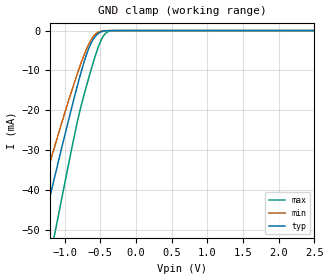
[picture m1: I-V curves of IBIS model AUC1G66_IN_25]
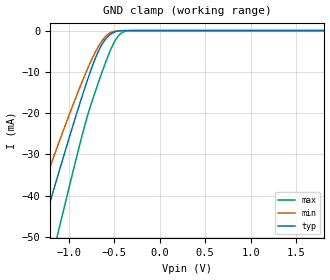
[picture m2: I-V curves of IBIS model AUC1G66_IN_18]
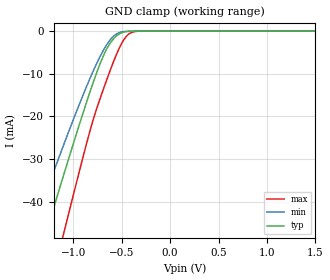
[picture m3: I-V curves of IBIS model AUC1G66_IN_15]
| TEXAS INSTRUMENTS INCORPORATED
| Standard Linear and Logic Group
| IBIS Model of SN74AUC1G66
| SINGLE BILATERAL ANALOG SWITCH
| This file contains package information for the following:
|  SOT 5-pin (DBV) package as [Component] AUC1G66_DBV
|  SOT 5-pin (DCK) package as [Component] AUC1G66_DCK
|  NanoStar WCSP 5-pin (YEA) package as [Component] AUC1G66_YEA
|  NanoFree WCSP 5-pin (YZA) package as [Component] AUC1G66_YZA
| This device can be powered at the following Vccs:
|  2.5 volt Vcc
|  1.8 volt Vcc
|  1.5 volt Vcc
|  1.2 volt Vcc
| This file provides unique models under the [Model Selector] for each Vcc.
| For operation at a specific Vcc, select the appropriate model after each
| [Model Selector] keyword.
[IBIS Ver]   3.2
[Comment char]  |_char
[File Name]   sn74auc1g66.ibs
[File Rev]   1.1 | x_die
[Date]   March 18, 2003
[Source]   Data created from TI-SPICE simulations at TI-SLL.
[Notes]   The following is an IBIS list for the SN74AUC1G66.
   Please contact sllibis@ti.com with questions and
   comments concerning SLL IBIS models.
   - Non-monotonic data due to FET characteristics.
   - C_comp values are taken at a different test condition than
   the Ci/Cio in data sheet.
   - Power-clamp data has been deleted from the input model
   since there is no power-clamp diode.
[Disclaimer] Property of Texas Instruments Incorporated. Unauthorized
   reproduction and/or distribution is strictly prohibited.
   This product is protected under copyright law.
   Created 2003,(C) Copyright 2003, Texas Instruments
   Incorporated, All Rights Reserved
   UNLESS THERE IS A SIGNED, WRITTEN AGREEMENT TO THE
   CONTRARY, TEXAS INSTRUMENTS (TI) IS PROVIDING THE IBIS
   MODELS AND WITHOUT ANY WARRANTY, EXPRESSED OR
   IMPLIED. TI assumes no liability for:
   1) the accuracy of the IBIS models provided to your
   company;
   2) the proper functioning of these IBIS Models in your
   design or for any resulting applications; or
   3) infringement of patents, copyrights or intellectual
   property rights resulting from your use of these IBIS
   models.
   TI provides IBIS Models as a service to our customers.
   You and your company shall not distribute, sell or give
   these models to anyone else without prior written
   permission from TI.
   TI reserves the right to make changes to our products or
   to discontinue any semiconductor product or service
   without notice, and advises our customers to obtain the
   latest version of relevant information to verify, before
   placing orders, that the information being relied on is
   current.
   Please be aware that your receipt and use of the IBIS
   information provided shall serve as acceptance of these
   terms and conditions. If you do not accept these terms,
   you should return or destroy the IBIS models and any
   other accompanying information immediately.
| Component AUC1G66_DBV 5-pin SOT
[Component]   AUC1G66_DBV
[Manufacturer]   Texas Instruments, Inc.
[Package]
|   typ   min   max
R_pkg   2.500e-02   2.100e-02   2.900e-02
L_pkg   1.529e-09   1.312e-09   1.906e-09
C_pkg   1.560e-13   1.100e-13   2.400e-13
[Pin]   signal_name   model_name   R_pin   L_pin   C_pin
1   A   AUC1G66_IO   2.100e-02   1.511e-09   1.440e-13
2   B   AUC1G66_IO   2.300e-02   1.312e-09   1.380e-13
3   GND   GND   2.900e-02   1.906e-09   2.400e-13
4   C   AUC1G66_IN   2.600e-02   1.541e-09   1.500e-13
5   VCC   POWER   2.500e-02   1.374e-09   1.100e-13
| Component AUC1G66_DCK 5-pin SOT
[Component]   AUC1G66_DCK
[Manufacturer]   Texas Instruments, Inc.
[Package]
|   typ   min   max
R_pkg   2.000e-02   1.700e-02   2.500e-02
L_pkg   9.980e-10   8.810e-10   1.069e-09
C_pkg   1.460e-13   1.180e-13   2.050e-13
[Pin]   signal_name   model_name   R_pin   L_pin   C_pin
1   A   AUC1G66_IO   1.900e-02   1.069e-09   1.620e-13
2   B   AUC1G66_IO   1.800e-02   8.810e-10   1.210e-13
3   GND   GND   1.700e-02   1.031e-09   2.050e-13
4   C   AUC1G66_IN   2.000e-02   9.600e-10   1.240e-13
5   VCC   POWER   2.500e-02   1.049e-09   1.180e-13
| Component AUC1G66_YEA 5-pin NanoStar WCSP
[Component]   AUC1G66_YEA
[Manufacturer]   Texas Instruments, Inc.
[Package]
|   typ   min   max
R_pkg   0.001   0.001   0.001
L_pkg   0.021nH   0.021nH   0.021nH
C_pkg   0.046pF   0.045pF   0.047pF
[Pin]   signal_name   model_name   R_pin   L_pin   C_pin
1   A   AUC1G66_IO   0.001   0.021nH   0.046pF
2   B   AUC1G66_IO   0.001   0.021nH   0.047pF
3   GND   GND   0.001   0.021nH   0.046pF
4   C   AUC1G66_IN   0.001   0.021nH   0.045pF
5   VCC   POWER   0.001   0.021nH   0.045pF
| Component AUC1G66_YZA 5-pin NanoFree WCSP
[Component]   AUC1G66_YZA
[Manufacturer]   Texas Instruments, Inc.
[Package]
|   typ   min   max
R_pkg   0.001   0.001   0.001
L_pkg   0.021nH   0.021nH   0.021nH
C_pkg   0.046pF   0.045pF   0.047pF
[Pin]   signal_name   model_name   R_pin   L_pin   C_pin
1   A   AUC1G66_IO   0.001   0.021nH   0.046pF
2   B   AUC1G66_IO   0.001   0.021nH   0.047pF
3   GND   GND   0.001   0.021nH   0.046pF
4   C   AUC1G66_IN   0.001   0.021nH   0.045pF
5   VCC   POWER   0.001   0.021nH   0.045pF
[Series Switch Groups]
| Function Group States
On  1 /   | A<->B(C=HIGH)
Off 1 /   | A<-x->B(C=LOW)
[Series Pin Mapping]   pin_2   model_name   function_table_group
1   2   AUC1G66_IO_25_S   1
| 1   2   AUC1G66_IO_18_S   1
| 1   2   AUC1G66_IO_15_S   1
| 1   2   AUC1G66_IO_12_S   1
| Model AUC1G66_IN
[Model Selector]   AUC1G66_IN
AUC1G66_IN_25   2.5 volt Vcc
AUC1G66_IN_18   1.8 volt Vcc
AUC1G66_IN_15   1.5 volt Vcc
AUC1G66_IN_12   1.2 volt Vcc
| Model AUC1G66_IO
[Model Selector]   AUC1G66_IO
AUC1G66_IO_25   2.5 volt Vcc
AUC1G66_IO_18   1.8 volt Vcc
AUC1G66_IO_15   1.5 volt Vcc
AUC1G66_IO_12   1.2 volt Vcc
| Model AUC1G66_IO_S
[Model Selector]   AUC1G66_IO_S
AUC1G66_IO_25_S   2.5 volt Vcc
AUC1G66_IO_18_S   1.8 volt Vcc
AUC1G66_IO_15_S   1.5 volt Vcc
AUC1G66_IO_12_S   1.2 volt Vcc
[Model]   AUC1G66_IO_25_S
Model_type  Series_switch
| variable   typ   min   max
C_comp   0   0   0
[Temperature Range]   40   100   -40
| Ambient temperature   25   85   -40
[Voltage range]   2.5   2.3   2.7
[On]
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[Off]
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[Model]   AUC1G66_IO_18_S
Model_type  Series_switch
| variable   typ   min   max
C_comp   0   0   0
[Temperature Range]   40   100   -40
| Ambient temperature   25   85   -40
[Voltage range]   1.8   1.65   1.95
[On]
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[Off]
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[Model]   AUC1G66_IO_15_S
Model_type  Series_switch
| variable   typ   min   max
C_comp   0   0   0
[Temperature Range]   40   100   -40
| Ambient temperature   25   85   -40
[Voltage range]   1.5   1.4   1.6
[On]
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[Off]
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[Model]   AUC1G66_IO_12_S
Model_type  Series_switch
| variable   typ   min   max
C_comp   0   0   0
[Temperature Range]   40   100   -40
| Ambient temperature   25   85   -40
[Voltage range]   1.2   1.1   1.3
[On]
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[Off]
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| Models and submodels in the file (12): AUC1G66_IN_25 (Input), AUC1G66_IN_18 (Input), AUC1G66_IN_15 (Input), AUC1G66_IN_12 (Input), AUC1G66_IO_25_S (Series_switch), AUC1G66_IO_25 (Terminator), AUC1G66_IO_18_S (Series_switch), AUC1G66_IO_18 (Terminator), AUC1G66_IO_15_S (Series_switch), AUC1G66_IO_15 (Terminator), AUC1G66_IO_12_S (Series_switch), AUC1G66_IO_12 (Terminator)
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[Model]   AUC1G66_IN_25
Model_type  Input
Vinl=0.7
Vinh=1.7
| variable   typ   min   max
C_comp   1.89pF   1.48pF   2.30pF
[Temperature Range]   40   100   -40
| Ambient temperature   25   85   -40
[Voltage range]   2.5   2.3   2.7
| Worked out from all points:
|   GND clamp passes 1 mA (typ) near -0.55 V on its own axis
[GND Clamp]
| AUC1G66_IN_25
|   Voltage   I(typ)   I(min)   I(max)
-2.7V     -157mA     -130.3mA   -191.7mA
-1.47V    -61.86mA   -49.74mA   -81.22mA
-1.32V    -50.42mA   -40.3mA    -67.62mA
-1.15V    -37.6mA    -29.81mA   -52.18mA
-1.11V    -34.62mA   -27.39mA   -48.55mA
-855mV    -16.2mA    -12.62mA   -25.76mA
-740mV    -8.694mA   -6.762mA   -17.01mA
-635mV    -3.435mA   -2.557mA   -10.25mA
-530mV    -751.7uA   -416uA     -4.264mA
-440mV    -95.44uA   -46.04uA   -977.4uA
-335mV    -4.571uA   -2.694uA   -44.25uA
2.5V      313.9pA    402pA      470.4pA
[Model]   AUC1G66_IN_18
Model_type  Input
Vinl=0.5775
Vinh=1.2675
| variable   typ   min   max
C_comp   1.97pF   1.57pF   2.31pF
[Temperature Range]   40   100   -40
| Ambient temperature   25   85   -40
[Voltage range]   1.8   1.65   1.95
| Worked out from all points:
|   GND clamp passes 1 mA (typ) near -0.55 V on its own axis
[GND Clamp]
| AUC1G66_IN_18
|   Voltage   I(typ)   I(min)   I(max)
-2.7V     -157mA     -130.3mA   -191.7mA
-1.485V   -63.01mA   -50.7mA    -82.58mA
-1.435V   -59.19mA   -47.53mA   -78.05mA
-1.295V   -48.52mA   -38.74mA   -65.35mA
-1.13V    -36.11mA   -28.6mA    -50.37mA
-1.09V    -33.13mA   -26.19mA   -46.74mA
-735mV    -8.396mA   -6.53mA    -16.67mA
-640mV    -3.626mA   -2.718mA   -10.56mA
-540mV    -904.5uA   -517.4uA   -4.766mA
-445mV    -108.7uA   -52.4uA    -1.09mA
-345mV    -6.234uA   -3.562uA   -63.03uA
1.8V      203.2pA    298.4pA    235.5pA
[Model]   AUC1G66_IN_15
Model_type  Input
Vinl=0.49
Vinh=1.04
| variable   typ   min   max
C_comp   2.01pF   1.62pF   2.32pF
[Temperature Range]   40   100   -40
| Ambient temperature   25   85   -40
[Voltage range]   1.5   1.4   1.6
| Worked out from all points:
|   GND clamp passes 1 mA (typ) near -0.55 V on its own axis
[GND Clamp]
| AUC1G66_IN_15
|   Voltage   I(typ)   I(min)   I(max)
-2.7V     -157mA     -130.3mA   -191.7mA
-1.45V    -60.33mA   -48.48mA   -79.41mA
-1.405V   -56.89mA   -45.63mA   -75.33mA
-1.27V    -46.63mA   -37.19mA   -63.08mA
-1.11V    -34.62mA   -27.39mA   -48.55mA
-1.075V   -32.02mA   -25.29mA   -45.38mA
-740mV    -8.694mA   -6.762mA   -17.01mA
-640mV    -3.626mA   -2.718mA   -10.56mA
-540mV    -904.5uA   -517.4uA   -4.766mA
-445mV    -108.7uA   -52.4uA    -1.09mA
-340mV    -5.34uA    -3.098uA   -52.88uA
1.5V      165.9pA    259.7pA    172.1pA
